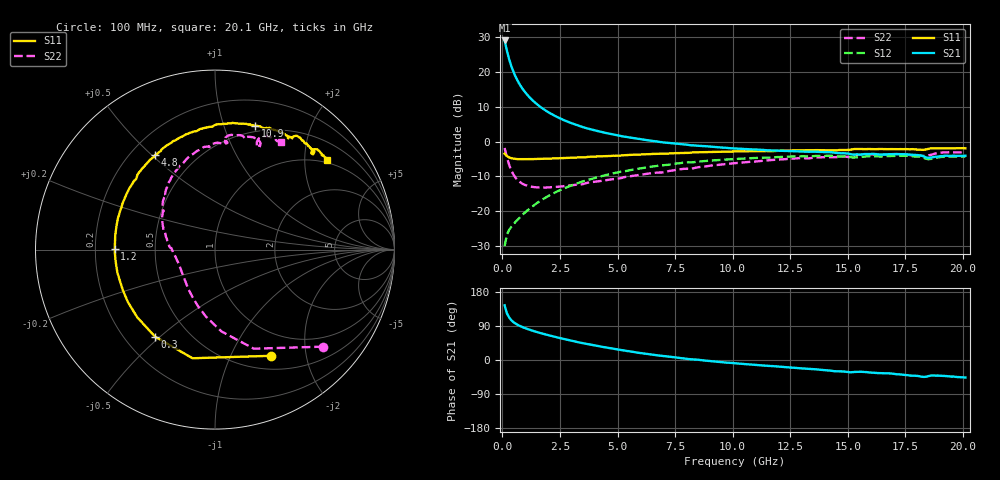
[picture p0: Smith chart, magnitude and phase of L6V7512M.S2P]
!  Infineon Technologies AG
! BFR380L3 , PF131585-7, No.6, Th 09.10.01, soldered on pcb-board, measured with PP GSG850
!  Vce=0.75 V,  Ic=12.5 mA
! Common Emitter S-Parameters:  15. November 2001
#  GHz  S  MA  R  50
! f  S11  S21  S12  S22
! GHz  Mag  Ang  Mag  Ang  Mag  Ang  Mag  Ang
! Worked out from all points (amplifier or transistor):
!   201 points, 100 MHz to 20.1 GHz, reference 50 ohm
!   highest |S21| = 29.1 dB at 100 MHz (marker M1)
!   |S21| within 3 dB of that: start of sweep to 203 MHz
!   unconditionally stable (mu >= 1): 1.548 GHz to 5.195 GHz; 18.3 GHz to 18.53 GHz
!   at 3.4 GHz: K = 1.03, MAG = 6.9 dB, |S12| = -11.7 dB
!   at 10.1 GHz: K = 0.98, MSG = 1.5 dB, |S12| = -5.0 dB
!   at 20.1 GHz: K = 0.99, MSG = 0.1 dB, |S12| = -4.3 dB
!   S11 on the Smith chart (normalised r, x): 100 MHz: 0.67, -1.43; 300 MHz: 0.32, -0.48; 1.2 GHz: 0.28, +0.00; 4.8 GHz: 0.30, +0.51; 10.9 GHz: 0.44, +1.28; 20.1 GHz: 0.94, +2.57
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0.1  0.668 -62.3  28.53 144.4  0.03114 61.7  0.8085 -42.0
0.2  0.6182 -101.7  20.38 123.4  0.04566 51.2  0.593 -68.6
0.3  0.5889 -124.6  15.17 111.8  0.05365 47.6  0.4578 -85.4
0.4  0.5744 -138.9  11.93 104.4  0.05953 47.1  0.3771 -97.7
0.5  0.5666 -148.9  9.764 99.1  0.06508 48.4  0.3269 -107.2
0.6  0.561 -156.2  8.248 95.1  0.07123 49.8  0.2942 -115.0
0.7  0.5578 -162.0  7.143 91.7  0.07701 51.2  0.2717 -121.7
0.8  0.5586 -166.9  6.287 88.7  0.08299 52.5  0.2557 -127.3
0.9  0.5575 -170.9  5.62 86.2  0.08949 53.7  0.244 -132.2
1  0.5574 -174.4  5.085 83.8  0.09585 54.7  0.236 -136.5
1.2  0.5584 179.5  4.271 79.5  0.1092 56.0  0.2258 -143.6
1.6  0.5621 169.9  3.253 72.0  0.1367 57.2  0.2178 -154.4
2.1  0.5686 160.2  2.526 63.9  0.1714 56.8  0.2195 -164.0
2.7  0.579 150.2  2.015 55.0  0.2127 54.6  0.2288 -173.0
3.5  0.5897 138.3  1.613 44.4  0.2671 50.4  0.2434 178.0
4.8  0.6242 122.2  1.266 29.8  0.347 42.3  0.2869 163.6
6.8  0.6661 101.3  0.9932 11.8  0.4502 28.6  0.3582 143.7
10.1  0.72 76.7  0.7932 -8.7  0.5599 7.6  0.4886 116.8
10.9  0.7264 72.1  0.7679 -12.4  0.5774 2.8  0.5131 110.3
13.5  0.7495 59.7  0.7145 -24.1  0.6158 -12.2  0.5831 92.3
16.8  0.7777 47.5  0.6578 -35.3  0.6174 -27.2  0.656 73.3
20.1  0.7993 38.4  0.6242 -46.1  0.6102 -40.3  0.7017 58.3
